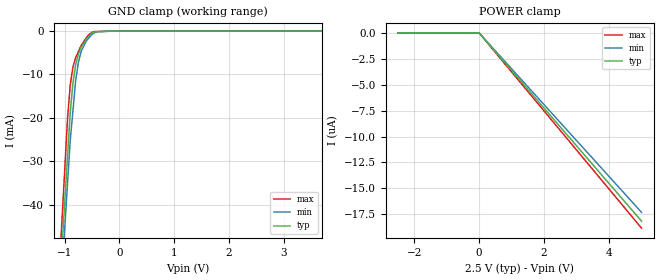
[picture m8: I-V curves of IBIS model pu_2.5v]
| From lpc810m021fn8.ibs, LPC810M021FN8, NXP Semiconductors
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[Model] pu_2.5v
Model_type Input
Vinl = 750.000mV
Vinh = 1.75000V
C_comp 909.000fF 904.000fF 914.000fF
| variable typ   min   max
[Voltage Range] 2.50000V 2.25000V 2.75000V
[POWER Clamp Reference] 2.50000V 2.25000V 2.75000V
[GND Clamp Reference] 0.00000V 0.00000V 0.00000V
[Temperature Range]   25   85   -40
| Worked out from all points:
|   GND clamp passes 1 mA (typ) near -0.54 V on its own axis
[GND Clamp]
-2.5V     -349.8mA   -345.7mA   -378.6mA
-950mV    -29.07mA   -35.25mA   -20.26mA
-900mV    -18.72mA   -25.23mA   -12.43mA
-850mV    -11.92mA   -18.26mA   -8.272mA
-800mV    -7.671mA   -11.29mA   -6.085mA
-750mV    -5.233mA   -7.175mA   -4.695mA
-700mV    -3.729mA   -4.674mA   -3.305mA
-600mV    -1.779mA   -2.158mA   -1.401mA
-500mV    -508.2uA   -753.7uA   -281.2uA
-400mV    -162.5uA   -132.2uA   -88.55uA
0V        0A         0A         0A
5V        0A         0A         0A
[POWER Clamp]
-2.5V     0A         0A         0A
0V        0A         0A         0A
5V        -18.17uA   -17.32uA   -18.84uA
